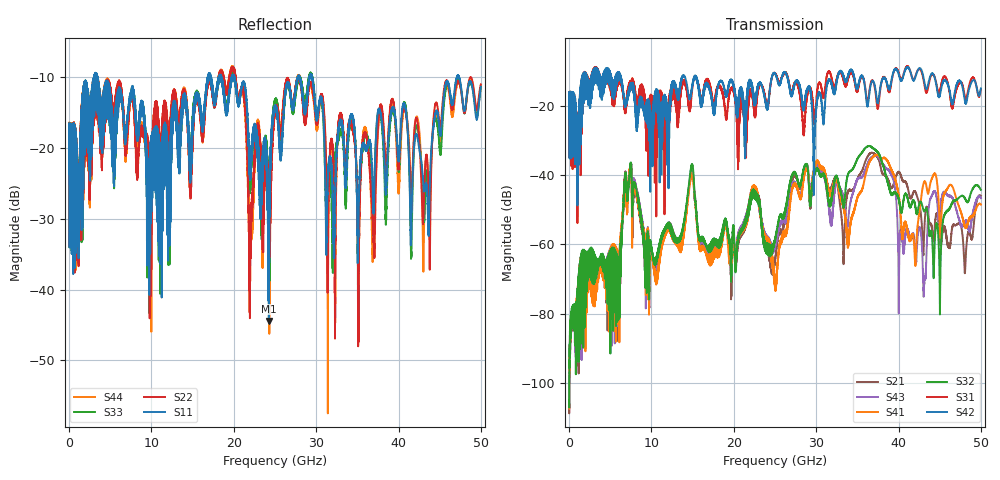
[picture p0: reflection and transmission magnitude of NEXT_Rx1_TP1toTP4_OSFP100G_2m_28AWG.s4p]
! Touchstone data
! Created: 27-Feb-2019 by IdEM 12 (12.1.0)
! COMMENTS
!  Created Wed Feb 27 12:03:36 2019
!  64 Port Network Data from SP1.SP block
!  freq  magS1_1  angS1_1  magS1_2  angS1_2  magS1_3  angS1_3  magS1_4  angS1_4
!  magS1_5  angS1_5  magS1_6  angS1_6  magS1_7  angS1_7  magS1_8  angS1_8
!  magS1_9  angS1_9  magS1_10  angS1_10  magS1_11  angS1_11  magS1_12  angS1_12
!  magS1_13  angS1_13  magS1_14  angS1_14  magS1_15  angS1_15  magS1_16  angS1_16
!  magS1_17  angS1_17  magS1_18  angS1_18  magS1_19  angS1_19  magS1_20  angS1_20
!  magS1_21  angS1_21  magS1_22  angS1_22  magS1_23  angS1_23  magS1_24  angS1_24
!  magS1_25  angS1_25  magS1_26  angS1_26  magS1_27  angS1_27  magS1_28  angS1_28
!  magS1_29  angS1_29  magS1_30  angS1_30  magS1_31  angS1_31  magS1_32  angS1_32
!  magS1_33  angS1_33  magS1_34  angS1_34  magS1_35  angS1_35  magS1_36  angS1_36
!  magS1_37  angS1_37  magS1_38  angS1_38  magS1_39  angS1_39  magS1_40  angS1_40
!  magS1_41  angS1_41  magS1_42  angS1_42  magS1_43  angS1_43  magS1_44  angS1_44
!  magS1_45  angS1_45  magS1_46  angS1_46  magS1_47  angS1_47  magS1_48  angS1_48
!  magS1_49  angS1_49  magS1_50  angS1_50  magS1_51  angS1_51  magS1_52  angS1_52
!  magS1_53  angS1_53  magS1_54  angS1_54  magS1_55  angS1_55  magS1_56  angS1_56
!  magS1_57  angS1_57  magS1_58  angS1_58  magS1_59  angS1_59  magS1_60  angS1_60
!  magS1_61  angS1_61  magS1_62  angS1_62  magS1_63  angS1_63  magS1_64  angS1_64
!  magS2_1  angS2_1  magS2_2  angS2_2  magS2_3  angS2_3  magS2_4  angS2_4
!  magS2_5  angS2_5  magS2_6  angS2_6  magS2_7  angS2_7  magS2_8  angS2_8
!  magS2_9  angS2_9  magS2_10  angS2_10  magS2_11  angS2_11  magS2_12  angS2_12
!  magS2_13  angS2_13  magS2_14  angS2_14  magS2_15  angS2_15  magS2_16  angS2_16
!  magS2_17  angS2_17  magS2_18  angS2_18  magS2_19  angS2_19  magS2_20  angS2_20
!  magS2_21  angS2_21  magS2_22  angS2_22  magS2_23  angS2_23  magS2_24  angS2_24
!  magS2_25  angS2_25  magS2_26  angS2_26  magS2_27  angS2_27  magS2_28  angS2_28
!  magS2_29  angS2_29  magS2_30  angS2_30  magS2_31  angS2_31  magS2_32  angS2_32
!  magS2_33  angS2_33  magS2_34  angS2_34  magS2_35  angS2_35  magS2_36  angS2_36
!  magS2_37  angS2_37  magS2_38  angS2_38  magS2_39  angS2_39  magS2_40  angS2_40
!  magS2_41  angS2_41  magS2_42  angS2_42  magS2_43  angS2_43  magS2_44  angS2_44
!  magS2_45  angS2_45  magS2_46  angS2_46  magS2_47  angS2_47  magS2_48  angS2_48
!  magS2_49  angS2_49  magS2_50  angS2_50  magS2_51  angS2_51  magS2_52  angS2_52
!  magS2_53  angS2_53  magS2_54  angS2_54  magS2_55  angS2_55  magS2_56  angS2_56
!  magS2_57  angS2_57  magS2_58  angS2_58  magS2_59  angS2_59  magS2_60  angS2_60
!  magS2_61  angS2_61  magS2_62  angS2_62  magS2_63  angS2_63  magS2_64  angS2_64
!  magS3_1  angS3_1  magS3_2  angS3_2  magS3_3  angS3_3  magS3_4  angS3_4
!  magS3_5  angS3_5  magS3_6  angS3_6  magS3_7  angS3_7  magS3_8  angS3_8
!  magS3_9  angS3_9  magS3_10  angS3_10  magS3_11  angS3_11  magS3_12  angS3_12
!  magS3_13  angS3_13  magS3_14  angS3_14  magS3_15  angS3_15  magS3_16  angS3_16
!  magS3_17  angS3_17  magS3_18  angS3_18  magS3_19  angS3_19  magS3_20  angS3_20
!  magS3_21  angS3_21  magS3_22  angS3_22  magS3_23  angS3_23  magS3_24  angS3_24
!  magS3_25  angS3_25  magS3_26  angS3_26  magS3_27  angS3_27  magS3_28  angS3_28
!  magS3_29  angS3_29  magS3_30  angS3_30  magS3_31  angS3_31  magS3_32  angS3_32
!  magS3_33  angS3_33  magS3_34  angS3_34  magS3_35  angS3_35  magS3_36  angS3_36
!  magS3_37  angS3_37  magS3_38  angS3_38  magS3_39  angS3_39  magS3_40  angS3_40
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# Hz S MA R 50
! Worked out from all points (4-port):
!   5000 points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, 10 MHz to 50 GHz, reference 50 ohm
!   strongest paths, dB at 10 MHz, 12.51 GHz, 25.01 GHz, 37.51 GHz, 50 GHz:
!     S42: -18.0, -13.6, -10.8, -19.3, -15.1
!     S31: -18.0, -15.9, -10.7, -20.7, -15.4
!     S32: -104.8, -57.3, -58.9, -33.6, -44.3
!     S41: -105.8, -57.7, -70.5, -34.3, -48.5
!     S43: -106.0, -56.8, -60.6, -34.7, -46.6
!     S21: -105.8, -57.9, -64.9, -35.2, -46.0
!   lowest |S11| = -44.4 dB at 24.26 GHz (marker M1), VSWR 1.01, Z = 49.6 - j0.401 ohm
!   |S11| at or under -10 dB: 3.451 GHz to 16.86 GHz (13.4 GHz wide, 132 % of centre); 20.09 GHz to 27.79 GHz (7.695 GHz wide, 32.1 % of centre); 29.5 GHz to 47.1 GHz (17.61 GHz wide, 46 % of centre)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
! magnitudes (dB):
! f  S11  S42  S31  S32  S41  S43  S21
! 10 MHz  -17.7  -18.0  -18.0  -104.8  -105.8  -106.0  -105.8
! 7.39 GHz  -12.7  -14.9  -14.3  -39.0  -38.5  -38.7  -38.6
! 10.56 GHz  -23.8  -18.2  -26.1  -64.1  -68.6  -68.0  -65.6
! 14.88 GHz  -20.2  -15.2  -17.2  -37.3  -39.9  -38.4  -38.5
! 24.26 GHz  -44.4  -17.7  -18.3  -63.2  -60.3  -60.5  -63.8
! 28.77 GHz  -13.9  -16.8  -19.8  -36.8  -38.4  -37.9  -37.0
! 50 GHz  -11.4  -15.1  -15.4  -44.3  -48.5  -46.6  -46.0
